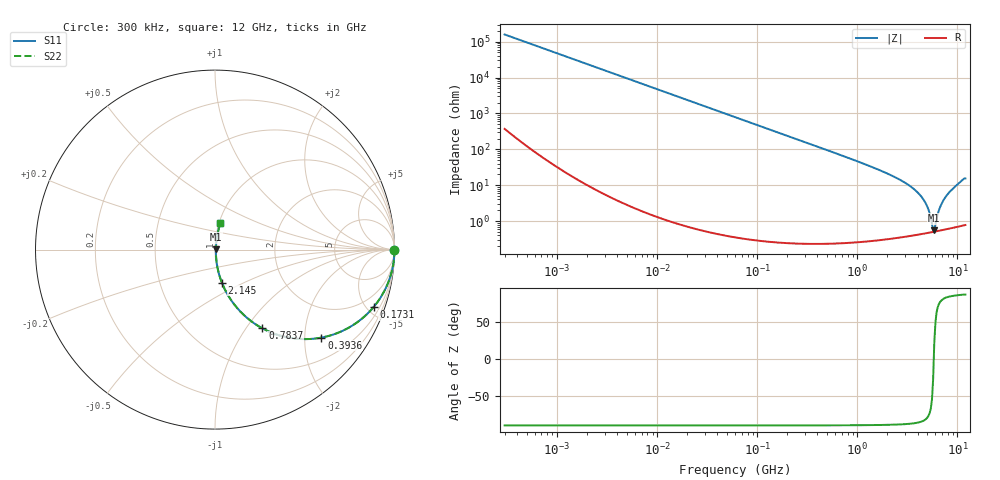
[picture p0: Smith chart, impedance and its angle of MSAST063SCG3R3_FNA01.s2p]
! MSAST063SCG3R3_FNA01  S-PARAMETER MODEL  ( Standard Model )
! Model Generated by TAIYO YUDEN Corporation (http://www.ty-top.com)
! Version 1.0
! TAIYO YUDEN Control No. 241122
! Copyright(c) 2024 TAIYO YUDEN CO.,LTD. All Rights Reserved.
! Product Description (link to TY-COMPAS)
! https://ds.yuden.co.jp/TYCOMPAS/or/detail?pn=MSAST063SCG3R3CFNA01&u=M
! Products Name : Multilayer Ceramic Capacitors
! Characteristics :
!  Capacitance : 3.3 [pF] , Rated Voltage : 25 [V] , TCC : CG / C0G
!  Case Size : 0.6 x 0.3 / 0.024 x 0.012 [mm/inch] , Thickness : 0.3 / 0.012 [mm/inch]
!  (Conditions: Temperature = 25 [degC] , DC Bias Voltage = 0 [V])
! External Node Assignments :
!  1  o---| |---o  2
! GND o---------o GND
! Frequency Range : 0.3MHz  -  12000MHz  [ 401 STEP ]
# MHZ S RI R 50
! Freq[MHz].  S11 Real  S11 Imag  S21 Real  S21 Imag  S12 Real  S12 Imag  S22 Real  S22 Imag
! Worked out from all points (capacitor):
!   401 points, 300 kHz to 12 GHz, reference 50 ohm
!   read as one part in series: C = 3.34 pF near 316.3 kHz
!   lowest |Z| = 545 mohm at 5.869 GHz (marker M1)
!   series resonance near 5.8 GHz, so ESL is about 230 pH
!   S11 on the Smith chart (normalised r, x): 300 kHz: open; 173.1 MHz: 1.00, -5.51; 393.6 MHz: 1.00, -2.41; 783.7 MHz: 1.00, -1.20; 2.145 GHz: 1.01, -0.38; 12 GHz: 1.02, +0.31
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0.3  1 -0.000629  1.86e-06 0.000629  1.86e-06 0.000629  1 -0.000629
1.769972  1 -0.00371  1.54e-05 0.00371  1.54e-05 0.00371  1 -0.00371
10.44266  0.9995 -0.0219  0.000485 0.0219  0.000485 0.0219  0.9995 -0.0219
60  0.9844 -0.1238  0.0156 0.1238  0.0156 0.1238  0.9844 -0.1238
173.124  0.8833 -0.3206  0.1167 0.3206  0.1167 0.3206  0.8833 -0.3206
353.9943  0.6431 -0.4782  0.3569 0.4782  0.3569 0.4782  0.6431 -0.4782
393.5654  0.5927 -0.4904  0.4073 0.4904  0.4073 0.4904  0.5927 -0.4904
783.7017  0.2641 -0.4388  0.7359 0.4388  0.7359 0.4388  0.2641 -0.4388
1229.528  0.1226 -0.3244  0.8774 0.3244  0.8774 0.3244  0.1226 -0.3244
2088.533  0.0409 -0.1902  0.9591 0.1902  0.9591 0.1902  0.0409 -0.1902
2144.601  0.0384 -0.1842  0.9616 0.1842  0.9616 0.1842  0.0384 -0.1842
3190.978  0.0144 -0.1025  0.9856 0.1025  0.9856 0.1025  0.0144 -0.1025
4158.869  0.00728 -0.0552  0.9927 0.0552  0.9927 0.0552  0.00728 -0.0552
4875.354  0.00537 -0.0286  0.9946 0.0286  0.9946 0.0286  0.00537 -0.0286
5140.631  0.00507 -0.0198  0.9949 0.0198  0.9949 0.0198  0.00507 -0.0198
5565.855  0.00492 -0.00685  0.9951 0.00685  0.9951 0.00685  0.00492 -0.00685
5868.704  0.00502 0.00204  0.995 -0.00204  0.995 -0.00204  0.00502 0.00204
6026.253  0.00513 0.00584  0.9949 -0.00584  0.9949 -0.00584  0.00513 0.00584
6699.894  0.00594 0.0233  0.9941 -0.0233  0.9941 -0.0233  0.00594 0.0233
7648.807  0.00807 0.0472  0.9919 -0.0472  0.9919 -0.0472  0.00807 0.0472
9454.42  0.0146 0.0889  0.9854 -0.0889  0.9854 -0.0889  0.0146 0.0889
12000  0.0303 0.1479  0.9697 -0.1479  0.9697 -0.1479  0.0303 0.1479
